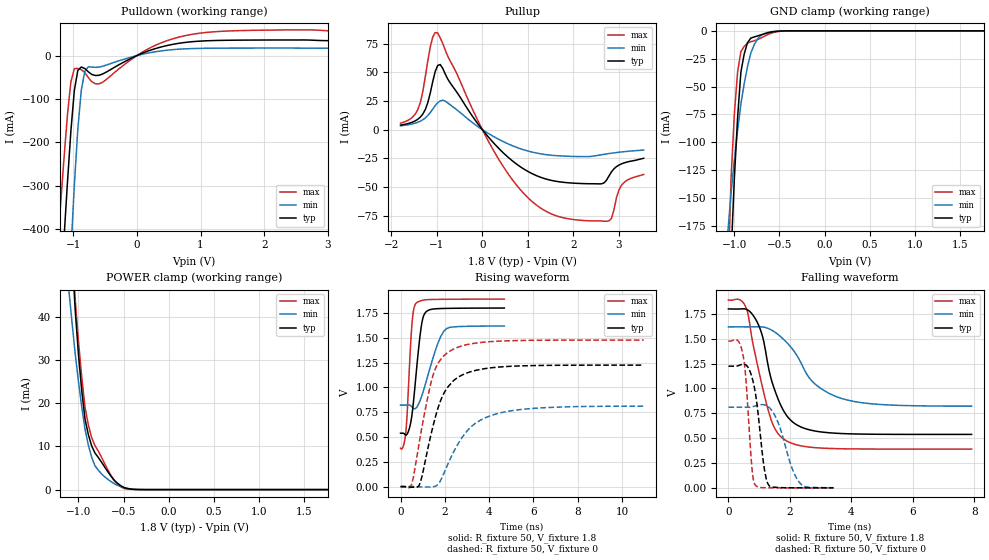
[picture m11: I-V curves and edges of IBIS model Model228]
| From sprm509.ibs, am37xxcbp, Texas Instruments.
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| Model based on original model for BQ18OMAPSMART2FBPB_SSBHH
|   Sub model T2FBPB_H_0_PUPD0_1P8
[model]   Model228
|[Input Load]   PI
|[Output Drive] LB0
|Voltage   1.8V
|Mode   I/O
Model_type   I/O
Polarity   Non-Inverting
Enable   Active-Low
Vinl =  0.63
Vinh =  1.17
Cref =  15pF
Rref =  100.0000M
Vref =  0V
Vmeas =  0.9
C_comp   1.612314p   1.445601p   1.775954p
[Model Spec]
Vinl   0.63   0.567   0.6615
Vinh   1.17   1.053   1.2285
[Temperature Range]   25   125   -40
[Voltage Range]   1.8   1.62   1.89
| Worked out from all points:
|   slope of the pulldown table from 0 to 0.27 V, typ, clamps not added: 17.8 ohm
|   slope of the pullup table from 0 to 0.27 V, typ, clamps not added: 21.5 ohm
|   GND clamp passes 1 mA (typ) near -0.58 V on its own axis
|   POWER clamp passes 1 mA (typ) near -0.54 V on its own axis
|   rising waveform, R_fixture 50, V_fixture 1.8: 20-80 % time 343ps typ, 660ps min, 213ps max; typ from 0.538 V to 1.8 V
|   rising waveform, R_fixture 50, V_fixture 0: 20-80 % time 957ps typ, 1.43ns min, 830ps max; typ from 0 V to 1.22 V
|   falling waveform, R_fixture 50, V_fixture 1.8: 20-80 % time 682ps typ, 1.19ns min, 662ps max; typ from 1.8 V to 0.538 V
|   falling waveform, R_fixture 50, V_fixture 0: 20-80 % time 280ps typ, 490ps min, 196ps max; typ from 1.22 V to 0 V
[POWER_clamp]
-1.8V     449.2mA    229.3mA    499.9mA
-1.109V   70.03mA    46.65mA    71.76mA
-1.073V   55.15mA    38.86mA    56.96mA
-1.036V   41.47mA    31.41mA    43.93mA
-1V       31.2mA     24.93mA    34.21mA
-963.6mV  22.8mA     19.1mA     25.91mA
-927.3mV  16.27mA    13.92mA    19.01mA
-890.9mV  12.72mA    10.32mA    14.97mA
-818.2mV  8.506mA    5.529mA    10.22mA
-600mV    2.086mA    1.321mA    1.925mA
-381.8mV  46uA       75.05uA    15.45uA
1.764V    -1.718nA   -102nA     -1.848nA
[Pulldown]
-1.8V     -1.866A    -2.926A    -1.473A
-1.255V   -690.3mA   -1.165A    -458.8mA
-1.2V     -556.9mA   -981.3mA   -347.5mA
-1.145V   -424mA     -799.3mA   -238.7mA
-1.036V   -174.1mA   -452.5mA   -60.31mA
-981.8mV  -80.13mA   -298.3mA   -30.04mA
-872.7mV  -26.27mA   -79.78mA   -32.44mA
-763.6mV  -37.26mA   -25.87mA   -50.47mA
-545.5mV  -42.85mA   -24.82mA   -62.02mA
163.6mV   9.905mA    5.464mA    14.49mA
872.7mV   32.06mA    16.22mA    49.12mA
3.545V    34.18mA    16.99mA    56.07mA
[Pullup]
-1.8V     4.02mA     3.353mA    5.71mA
-1.418V   9.153mA    6.524mA    17.71mA
-1.255V   17.65mA    10.28mA    46.45mA
-1.091V   42.12mA    17.99mA    80.97mA
-981.8mV  56.04mA    23.5mA     84.34mA
-818.2mV  48.72mA    25.01mA    69.63mA
272.7mV   -12.68mA   -6.535mA   -20.08mA
1.255V    -41.13mA   -20.87mA   -67.69mA
2.564V    -47.26mA   -22.22mA   -79.57mA
2.782V    -40.42mA   -20.82mA   -79.47mA
3.055V    -29.85mA   -19.43mA   -48.72mA
3.545V    -24.9mA    -17.8mA    -39.06mA
[GND_clamp]
-1.8V     -3.26A     -1.496A    -3.636A
-1.073V   -295.4mA   -181.3mA   -234.2mA
-1.036V   -202.1mA   -145.8mA   -132.5mA
-1V       -132.6mA   -116.1mA   -74.83mA
-963.6mV  -77.56mA   -89.36mA   -36.83mA
-927.3mV  -36.94mA   -65.52mA   -18.53mA
-890.9mV  -20.86mA   -47.5mA    -14.02mA
-854.5mV  -10.73mA   -32.34mA   -11.09mA
-818.2mV  -6.545mA   -20.02mA   -9.764mA
-709.1mV  -3.764mA   -4.146mA   -6.62mA
-563.6mV  -769uA     -544.8uA   -1.476mA
1.764V    -70.42pA   812.3nA    3.348nA
[Ramp]
dV/dt_f  0.7587224/0.6815725n   0.47975/1.199481n   0.9054366/0.6649802n
dV/dt_r  0.7390167/0.9581515n  0.4899643/1.441589n   0.8941395/0.8323858n
R_load = 50
[Rising Waveform]
R_fixture = 50
V_fixture = 1.8
V_fixture_min = 1.62
V_fixture_max = 1.89
0s        537.7mV    821mV      387.2mV
126ps     537.8mV    821.3mV    407.9mV
243ps     518.1mV    820.9mV    556mV
504ps     703mV      805.3mV    1.604V
684ps     1.087V     788.5mV    1.844V
963ps     1.65V      916.6mV    1.876V
1.17ns    1.765V     1.069V     1.884V
1.701ns   1.794V     1.453V     1.887V
2.07ns    1.796V     1.591V     1.888V
4.689ns   1.799V     1.618V     1.89V
[Rising Waveform]
R_fixture = 50
V_fixture = 0
V_fixture_min = 0
V_fixture_max = 0
0s        -345.4uV   72.94uV    -1.174mV
450ps     -5.897mV   1.362mV    -5.757mV
585ps     -7.214mV   -43.54uV   99.93mV
837ps     10.22mV    -3.231mV   433mV
1.485ns   624.8mV    -2.071mV   1.134V
1.854ns   891mV      81.22mV    1.293V
2.259ns   1.035V     285.5mV    1.37V
3.159ns   1.157V     596.2mV    1.438V
4.383ns   1.204V     736.2mV    1.465V
10.98ns   1.224V     809.9mV    1.477V
[Falling Waveform]
R_fixture = 50
V_fixture = 1.8
V_fixture_min = 1.62
V_fixture_max = 1.89
0s        1.8V       1.62V      1.89V
351ps     1.8V       1.62V      1.895V
576ps     1.798V     1.62V      1.813V
918ps     1.678V     1.621V     1.274V
1.116ns   1.516V     1.619V     1.001V
1.413ns   1.072V     1.586V     664.9mV
1.89ns    729mV      1.465V     472.5mV
2.754ns   575.8mV    1.063V     406.5mV
3.69ns    546.6mV    898.7mV    393.5mV
7.911ns   537.9mV    822.8mV    390.2mV
[Falling Waveform]
R_fixture = 50
V_fixture = 0
V_fixture_min = 0
V_fixture_max = 0
0s        1.224V     811.6mV    1.476V
306ps     1.228V     811.9mV    1.482V
486ps     1.245V     811.7mV    1.318V
576ps     1.235V     811.4mV    1.062V
765ps     1.114V     815.1mV    198.5mV
873ps     960.8mV    824.2mV    27.7mV
1.179ns   169.4mV    835mV      1.643mV
1.332ns   18.25mV    806.9mV    986.7uV
2.322ns   483.3uV    49.65mV    211.6uV
3.42ns    124.8uV    1.648mV    50.57uV
